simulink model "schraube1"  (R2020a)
settings: Solver=VariableStepDiscrete  StartTime=0.0  StopTime=30  MaxStep=0.1  RelTol=1e-3  EnableMultiTasking=on
libraries: simulink x3

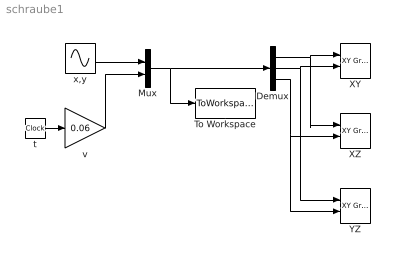
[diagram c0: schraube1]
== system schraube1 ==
  Demux : Demux  Outputs=3
  Mux : Mux  Inputs=2
  To Workspace : ToWorkspace  VariableName=schraub  SampleTime=-1
  XY : simulink/Sinks/XY Graph  xmin=-1.5  xmax=1.5  ymin=-1.5  ymax=1.5  st=-1
  XZ : simulink/Sinks/XY Graph  xmin=-1.5  xmax=1.5  ymin=-1  ymax=3  st=-1
  YZ : simulink/Sinks/XY Graph  xmin=-1.5  xmax=1.5  ymin=-1  ymax=3  st=-1
  t : Clock
  v : Gain  Gain=0.06
  x,y : Sin  Phase=[-pi/2, 0]  SampleTime=0
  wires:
  t/1 -> v/1
  x,y/1 -> Mux/1
  v/1 -> Mux/2
  Mux/1 -> To Workspace/1, Demux/1
  Demux/1 -> XY/1, XZ/1
  Demux/2 -> XY/2, YZ/1
  Demux/3 -> XZ/2, YZ/2
